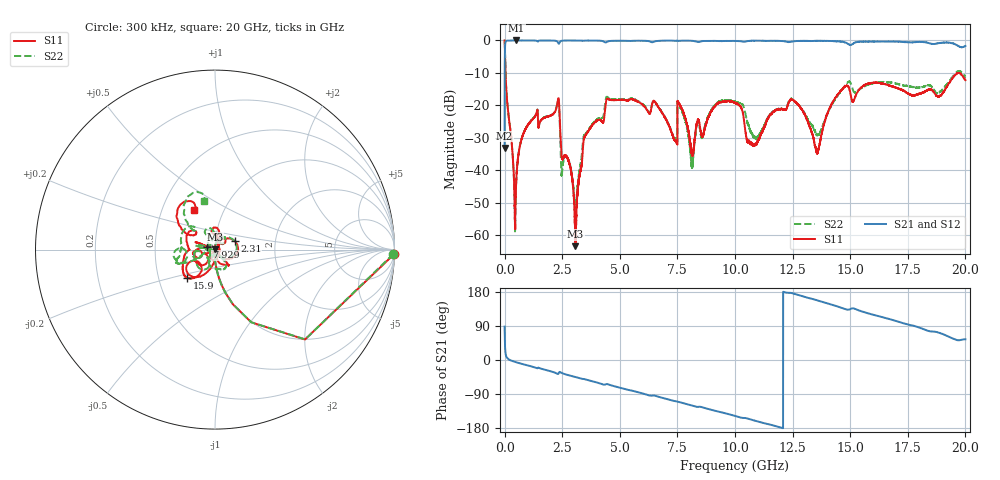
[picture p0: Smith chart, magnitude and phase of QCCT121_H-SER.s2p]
! Created Fri Feb  5 15:31:45 2021
# hz S ma R 50
! 2 Port Network Data from SP1.SP block
! freq  magS11  angS11  magS21  angS21  magS12  angS12  magS22  angS22
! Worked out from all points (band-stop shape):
!   20001 points, 300 kHz to 20 GHz, reference 50 ohm
!   highest |S21| = 0.00 dB at 510.3 MHz (marker M1); lowest = -33.1 dB at 300 kHz (marker M2)
!   |S21| within 3 dB of the highest: 13.47 MHz to end of sweep
!   lowest |S11| = -63.3 dB at 3.075 GHz (marker M3), VSWR 1.00, Z = 50 + j0.059 ohm
!   |S11| at or under -10 dB: 39.85 MHz to 19.68 GHz (19.64 GHz wide, 199 % of centre); 19.68295 GHz to 19.68673 GHz (3.78 MHz wide, 0.0192 % of centre); 19.75 GHz to end of sweep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
!   |S22| runs from -58.8 to 0.0 dB; largest |S21 - S12| = 0.015
!   S11 on the Smith chart (normalised r, x): 300 kHz: 8, -75; 2.31 GHz: 1.24, +0.12; 7.929 GHz: 0.91, +0.03; 15.9 GHz: 0.70, -0.23; 20 GHz: 0.73, +0.34
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300000  0.9971 -1.5  0.02223 88.1  0.02243 88.4  0.994 -1.4
1.073e8  0.1189 -84.8  0.9921 5.5  0.9922 5.5  0.1193 -84.8
5.103e8  0.007264 94.0  0.9995 -6.1  0.9969 -6.1  0.00747 93.4
9.453e8  0.04579 77.3  0.998 -13.4  0.9978 -13.4  0.04625 78.4
2.3103e9  0.1197 23.9  0.9393 -37.0  0.94 -37.0  0.1157 28.6
2.5093e9  0.01509 5.5  0.991 -35.0  0.9912 -35.0  0.01073 41.0
3.0753e9  0.0006839 120.3  0.9977 -45.0  0.9978 -45.0  0.002073 -37.5
3.3343e9  0.01166 -133.8  0.9926 -49.2  0.9929 -49.2  0.01559 -96.8
4.4903e9  0.1261 -150.4  0.9698 -64.3  0.9688 -64.2  0.1321 -138.8
6.6673e9  0.09517 177.3  0.9848 -96.7  0.9847 -96.7  0.09588 178.2
7.3983e9  0.02888 162.2  0.9877 -108.6  0.9884 -108.6  0.03117 -168.5
7.6003e9  0.1038 158.0  0.9874 -111.3  0.9882 -111.4  0.09705 164.6
7.9293e9  0.0493 162.5  0.9905 -116.8  0.9914 -116.8  0.04336 162.3
8.1373e9  0.01736 -147.6  0.9861 -120.4  0.9867 -120.4  0.01167 -134.8
8.3753e9  0.05892 -97.7  0.95 -123.8  0.9499 -123.7  0.05509 -91.1
1.00003e10  0.11 -51.1  0.9836 -147.5  0.9841 -147.6  0.1145 -73.9
1.07543e10  0.02544 -1.9  0.9882 -158.2  0.9895 -158.2  0.03552 -141.0
1.24553e10  0.1231 88.8  0.9604 176.7  0.9571 176.6  0.1257 107.6
1.33343e10  0.03851 58.1  0.9806 161.6  0.9802 161.5  0.05051 112.3
1.59013e10  0.2207 -135.1  0.9601 120.9  0.9623 121.1  0.2156 -158.9
1.66673e10  0.2046 -152.0  0.9608 108.4  0.9534 108.2  0.2263 -163.9
2e10  0.2455 118.0  0.8224 54.6  0.8151 54.5  0.2776 102.9
